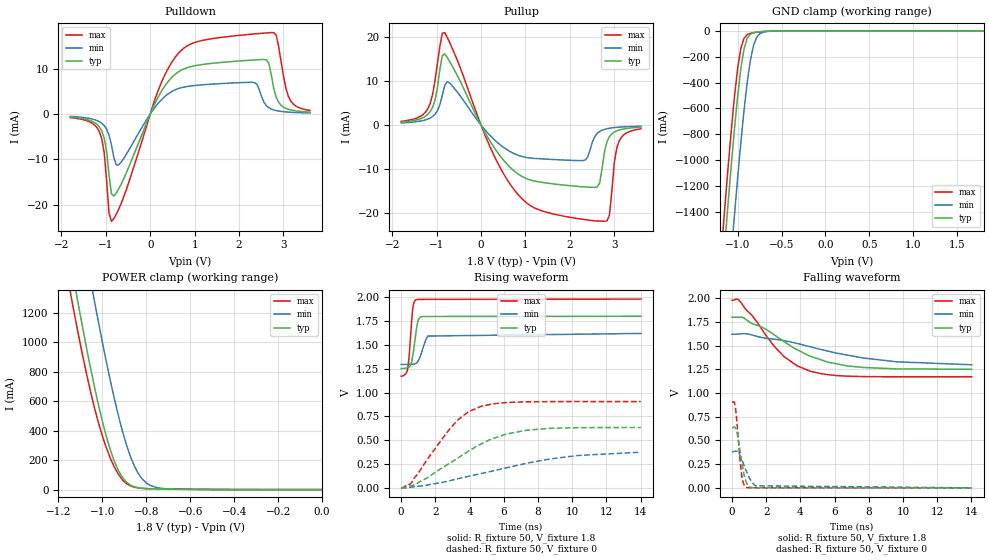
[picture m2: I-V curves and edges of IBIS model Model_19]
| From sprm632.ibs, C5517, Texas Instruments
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| Model based on original model for OC3350CT
|   Sub model OC3350CT_COM_1P8
[model]   Model_19
|[Description]  [1.8V-3-STATE-X-X]
|   , ,
|[Input Load]
|[Output Drive]
|Voltage   1.8V
|Mode   3-STATE
Model_type   3-state
Polarity   Non-Inverting
Enable   Active-Low
Cref =  15.0000pF
Rref =  100.0000M
Vref =  0V
Vmeas =  0.9
C_comp   1.382326p   1.3625191p   1.400048p
[Temperature Range]   25   105   -10
[Voltage Range]   1.8   1.62   1.98
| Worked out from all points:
|   slope of the pulldown table from 0 to 0.27 V, typ, clamps not added: 51 ohm
|   slope of the pullup table from 0 to 0.27 V, typ, clamps not added: 57.1 ohm
|   GND clamp passes 1 mA (typ) near -0.59 V on its own axis
|   POWER clamp passes 1 mA (typ) near -0.52 V on its own axis
|   rising waveform, R_fixture 50, V_fixture 1.8: 20-80 % time 259ps typ, 376ps min, 206ps max; typ from 1.25 V to 1.8 V
|   rising waveform, R_fixture 50, V_fixture 0: 20-80 % time 3.49ns typ, 5.74ns min, 2.29ns max; typ from 0.001 V to 0.634 V
|   falling waveform, R_fixture 50, V_fixture 1.8: 20-80 % time 3.24ns typ, 5.06ns min, 2.28ns max; typ from 1.8 V to 1.25 V
|   falling waveform, R_fixture 50, V_fixture 0: 20-80 % time 354ps typ, 550ps min, 263ps max; typ from 0.634 V to 0 V
[POWER_clamp]
-1.8V     7.656A     8.299A     7.406A
-1.145V   1.557A     2.196A     1.339A
-1.127V   1.405A     2.039A     1.195A
-1.109V   1.256A     1.883A     1.055A
-1.036V   703.1mA    1.284A     559.8mA
-981.8mV  361.6mA    868.9mA    284.1mA
-945.5mV  192.7mA    618.9mA    154mA
-909.1mV  83.65mA    400.5mA    67.92mA
-872.7mV  31.2mA     227.3mA    25.56mA
-818.2mV  8.542mA    72.07mA    8.371mA
-745.5mV  4.031mA    12.05mA    4.916mA
0V        133.9pA    2.238nA    111.9pA
[Pulldown]
-1.8V     -681.8uA   -528.3uA   -799.5uA
-1.145V   -2.847mA   -1.688mA   -3.913mA
-1.036V   -5.316mA   -2.553mA   -8.562mA
-872.7mV  -17.57mA   -6.854mA   -23.59mA
-709.1mV  -16.44mA   -11.17mA   -20.89mA
272.7mV   5.341mA    3.341mA    7.405mA
872.7mV   10.3mA     6.104mA    15.2mA
2.345V    11.88mA    6.92mA     17.61mA
2.618V    11.89mA    1.797mA    17.83mA
2.782V    5.623mA    889uA      17.88mA
3.109V    1.046mA    417.7uA    3.932mA
3.6V      416.6uA    227.7uA    789.5uA
[Pullup]
-1.8V     683.6uA    489.2uA    862.2uA
-1.2V     2.423mA    1.368mA    3.723mA
-818.2mV  16.21mA    9.062mA    21.1mA
218.2mV   -3.905mA   -2.516mA   -5.325mA
872.7mV   -11.39mA   -7.011mA   -16.27mA
2.345V    -14.1mA    -7.935mA   -21.55mA
2.618V    -14.08mA   -1.863mA   -21.85mA
2.782V    -5.911mA   -955uA     -21.92mA
2.891V    -2.622mA   -708.2uA   -20.54mA
3V        -1.581mA   -559.8uA   -8.602mA
3.109V    -1.114mA   -461.6uA   -3.637mA
3.6V      -465.3uA   -255.6uA   -860uA
[GND_clamp]
-1.8V     -7.797A    -8.487A    -7.522A
-1.182V   -1.972A    -2.683A    -1.686A
-1.145V   -1.654A    -2.361A    -1.372A
-1.109V   -1.345A    -2.044A    -1.067A
-1.036V   -766.4mA   -1.434A    -516.7mA
-1V       -510.9mA   -1.144A    -294.7mA
-963.6mV  -296.6mA   -871.1mA   -138.8mA
-927.3mV  -142.3mA   -620.2mA   -58.57mA
-890.9mV  -58.64mA   -401.5mA   -29.41mA
-818.2mV  -14.78mA   -112.1mA   -14.7mA
-709.1mV  -5.074mA   -10.31mA   -5.885mA
1.8V      133.9pA    3.271uA    -294.5pA
[Ramp]
dV/dt_f 0.33498681/3.2897334n 0.19919276/5.3081496n 0.49201805/2.3077935n
dV/dt_r 0.38059402/3.500797n  0.22885102/5.912113n  0.54384933/2.2938718n
R_load = 50
[Rising Waveform]
R_fixture = 50
V_fixture = 1.8
V_fixture_min = 1.62
V_fixture_max = 1.98
0s        1.252V     1.295V     1.172V
292.4ps   1.258V     1.296V     1.201V
395.5ps   1.261V     1.296V     1.267V
557.1ps   1.29V      1.297V     1.606V
675.6ps   1.381V     1.297V     1.874V
738.6ps   1.457V     1.299V     1.937V
869.4ps   1.636V     1.308V     1.973V
1.029ns   1.773V     1.342V     1.977V
1.55ns    1.798V     1.593V     1.978V
14.02ns   1.8V       1.62V      1.98V
[Rising Waveform]
R_fixture = 50
V_fixture = 0
V_fixture_min = 0
V_fixture_max = 0
0s        699.3uV    377.6uV    880.3uV
599.8ps   24.45mV    8.214mV    53.69mV
2.562ns   228mV      63.68mV    553.8mV
3.346ns   316.6mV    97.16mV    717.9mV
3.927ns   383.9mV    120.9mV    797.9mV
4.652ns   458.4mV    149.3mV    854.6mV
6.159ns   565.4mV    211.1mV    895.4mV
7.36ns    605.7mV    259.2mV    902.8mV
10.31ns   631.9mV    339.6mV    905.7mV
14.01ns   633.6mV    373.8mV    905.4mV
[Falling Waveform]
R_fixture = 50
V_fixture = 1.8
V_fixture_min = 1.62
V_fixture_max = 1.98
0s        1.8V       1.62V      1.98V
415.3ps   1.8V       1.623V     1.978V
1.854ns   1.686V     1.582V     1.644V
3.038ns   1.543V     1.553V     1.385V
3.805ns   1.458V     1.523V     1.287V
4.572ns   1.389V     1.488V     1.23V
5.625ns   1.325V     1.442V     1.194V
7.667ns   1.27V      1.37V      1.174V
9.634ns   1.255V     1.33V      1.171V
14.02ns   1.251V     1.299V     1.171V
[Falling Waveform]
R_fixture = 50
V_fixture = 0
V_fixture_min = 0
V_fixture_max = 0
0s        634mV      381.4mV    905.4mV
131.1ps   640.7mV    383.1mV    905.4mV
206.4ps   631.2mV    387.1mV    842.8mV
363.2ps   516.8mV    373.8mV    526.9mV
554.6ps   291.5mV    308mV      155.3mV
655.9ps   186.4mV    261.4mV    56.38mV
824.2ps   65.23mV    182mV      6.493mV
1.043ns   8.281mV    96.15mV    1.349mV
1.372ns   914.5uV    21.71mV    1.244mV
14.01ns   211.3nV    14.33uV    0V
